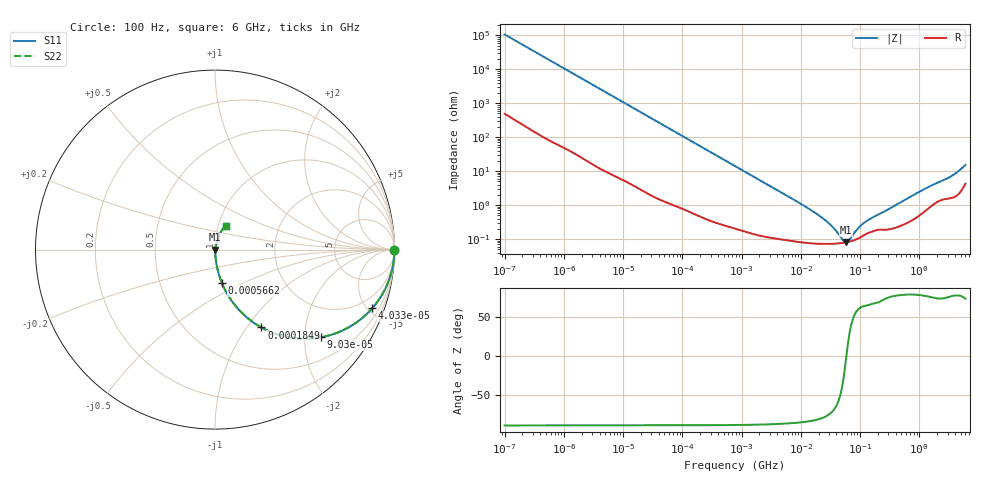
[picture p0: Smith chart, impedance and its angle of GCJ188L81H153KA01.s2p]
!Murata Part Number: GCJ188L81H153KA01
!These Parameters are Measured in Series Mode Connection
!Data Generated on Mar 13, 2026
!  o--ll--o
!Port1  Port2
!  o------o
!Operation Temp=25[degC], DC Bias Voltage=0[V]
!Freq. Start=100[Hz] Stop=6[GHz] 401[Steps]
# Hz S RI R 50
!Freq.(Hz) S11(Real) S11(Imag) S21(Real) S21(Imag) S12(Real) S12(Imag) S22(Real) S22(Imag)
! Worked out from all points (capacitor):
!   401 points, 100 Hz to 6 GHz, reference 50 ohm
!   read as one part in series: C = 15 nF near 109 Hz
!   lowest |Z| = 80.1 mohm at 56.99 MHz (marker M1)
!   series resonance near 58.83 MHz, so ESL is about 490 pH
!   S11 on the Smith chart (normalised r, x): 100 Hz: open; 40.34 kHz: 1.03, -5.36; 90.3 kHz: 1.02, -2.40; 184.9 kHz: 1.01, -1.18; 566.2 kHz: 1.00, -0.39; 6 GHz: 1.09, +0.29
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100  1 -0.000941  5.2e-06 0.000941  5.2e-06 0.000941  1 -0.000941
2008  0.9996 -0.0187  0.000437 0.0187  0.000437 0.0187  0.9996 -0.0187
11514  0.9882 -0.1055  0.0118 0.1055  0.0118 0.1055  0.9882 -0.1055
23569  0.9536 -0.2079  0.0464 0.2079  0.0464 0.2079  0.9536 -0.2079
40335  0.8765 -0.3262  0.1235 0.3262  0.1235 0.3262  0.8765 -0.3262
90302  0.5899 -0.4884  0.4101 0.4884  0.4101 0.4884  0.5899 -0.4884
184852  0.259 -0.434  0.741 0.434  0.741 0.434  0.259 -0.434
302498  0.1173 -0.317  0.8827 0.317  0.8827 0.317  0.1173 -0.317
566185  0.0381 -0.1853  0.9619 0.1853  0.9619 0.1853  0.0381 -0.1853
774597  0.0215 -0.1381  0.9785 0.1381  0.9785 0.1381  0.0215 -0.1381
2481164  0.00313 -0.0442  0.9969 0.0442  0.9969 0.0442  0.00313 -0.0442
1.555665e7  0.000787 -0.00671  0.9992 0.00671  0.9992 0.00671  0.000787 -0.00671
3.045065e7  0.000726 -0.0027  0.9993 0.0027  0.9993 0.0027  0.000726 -0.0027
5.211241e7  0.000772 -0.000464  0.9992 0.000464  0.9992 0.000464  0.000772 -0.000464
5.699437e7  0.000791 -0.000121  0.9992 0.000121  0.9992 0.000121  0.000791 -0.000121
6.518806e7  0.00083 0.000393  0.9992 -0.000393  0.9992 -0.000393  0.00083 0.000393
8.918374e7  0.001 0.00162  0.999 -0.00162  0.999 -0.00162  0.001 0.00162
1.166697e8  0.00131 0.0027  0.9987 -0.0027  0.9987 -0.0027  0.00131 0.0027
3.124326e8  0.00199 0.00759  0.998 -0.00759  0.998 -0.00759  0.00199 0.00759
1.251881e9  0.00743 0.0292  0.9926 -0.0292  0.9926 -0.0292  0.00743 0.0292
3.205649e9  0.0193 0.0615  0.9807 -0.0615  0.9807 -0.0615  0.0193 0.0615
6e9  0.0596 0.1319  0.9404 -0.1319  0.9404 -0.1319  0.0596 0.1319
